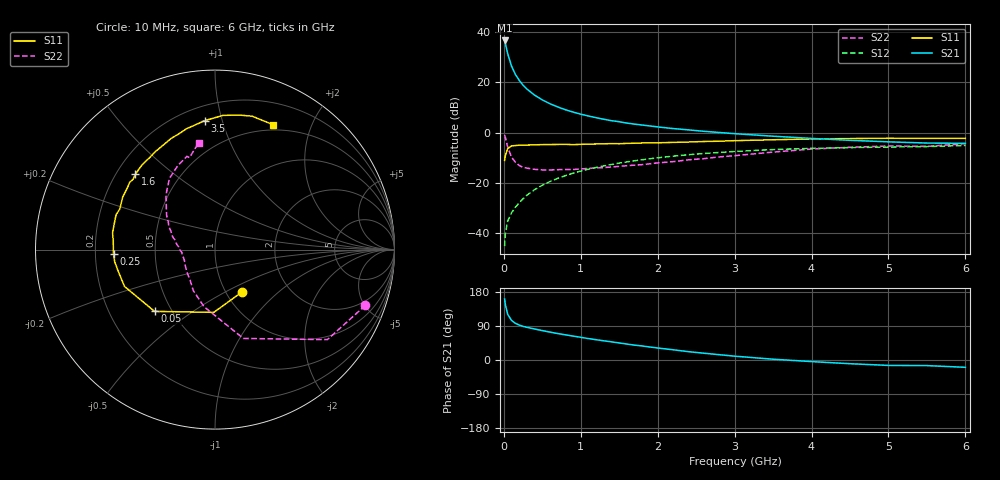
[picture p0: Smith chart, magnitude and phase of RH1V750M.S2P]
! SIEMENS Small Signal Semiconductors
! BFR106
! Si NPN RF Bipolar Junction Transistor in SOT23
! VCE = 1.75 V  IC = 50 mA
! Common Emitter S-Parameters:  August  1996
# GHz  S  MA  R  50
!  f  S11  S21  S12  S22
! GHz  MAG  ANG  MAG  ANG  MAG  ANG  MAG  ANG
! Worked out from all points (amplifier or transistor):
!   36 points, 10 MHz to 6 GHz, reference 50 ohm
!   highest |S21| = 36.7 dB at 10 MHz (marker M1)
!   |S21| within 3 dB of that: start of sweep to 33.3 MHz
!   unconditionally stable (mu >= 1): 223.2 MHz to 2.857 GHz; 4.977 GHz to end of sweep
!   at 250 MHz: K = 1.02, MAG = 21.7 dB, |S12| = -26.3 dB
!   at 1.4 GHz: K = 1.06, MAG = 7.2 dB, |S12| = -12.7 dB
!   at 6 GHz: K = 1.01, MAG = -0.2 dB, |S12| = -5.1 dB
!   S11 on the Smith chart (normalised r, x): 10 MHz: 1.19, -0.61; 50 MHz: 0.40, -0.36; 250 MHz: 0.28, -0.02; 1.6 GHz: 0.28, +0.37; 3.5 GHz: 0.29, +0.88; 6 GHz: 0.44, +1.48
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0.01  0.28 -57.0  68.26 161.0  0.0055 77.4  0.8932 -20.4
0.02  0.3497 -91.1  59.51 146.1  0.0099 68.7  0.8022 -38.7
0.05  0.4816 -134.4  37.21 120.5  0.0173 57.7  0.5195 -72.3
0.1  0.5446 -157.9  21.08 104.4  0.0254 59.7  0.3239 -100.9
0.15  0.553 -167.8  14.4 96.8  0.0326 63.5  0.2583 -118.0
0.2  0.5631 -173.1  10.99 92.3  0.0403 66.7  0.2211 -128.6
0.25  0.5658 -177.3  8.778 88.8  0.0484 68.0  0.2041 -138.3
0.3  0.5663 179.9  7.362 86.2  0.0569 69.5  0.1965 -144.1
0.4  0.5692 174.8  5.574 81.8  0.0733 70.5  0.1861 -153.8
0.5  0.5785 170.7  4.477 77.6  0.0897 70.2  0.181 -160.3
0.6  0.5786 166.9  3.754 73.6  0.1063 69.6  0.1806 -164.4
0.7  0.5816 163.2  3.25 69.8  0.1228 68.6  0.1832 -168.0
0.8  0.5841 160.5  2.856 66.4  0.1394 67.2  0.1849 -172.0
1.1  0.592 150.3  2.142 56.5  0.1874 63.1  0.1945 -179.1
1.3  0.5982 144.4  1.844 50.6  0.2182 59.7  0.2017 176.1
1.6  0.6108 136.5  1.548 42.1  0.2617 54.6  0.2196 170.4
2.2  0.6392 121.2  1.205 27.0  0.3402 44.4  0.2643 157.8
2.8  0.6752 107.4  1.007 14.0  0.403 34.2  0.3287 145.0
3.5  0.7209 94.5  0.849 2.1  0.4605 23.3  0.4099 131.8
4.5  0.7614 80.0  0.703 -9.8  0.5031 9.1  0.5108 114.1
5.5  0.7665 68.7  0.62 -14.8  0.5278 0.6  0.5319 105.5
6  0.7682 65.0  0.612 -19.3  0.5538 -6.1  0.6033 98.6
